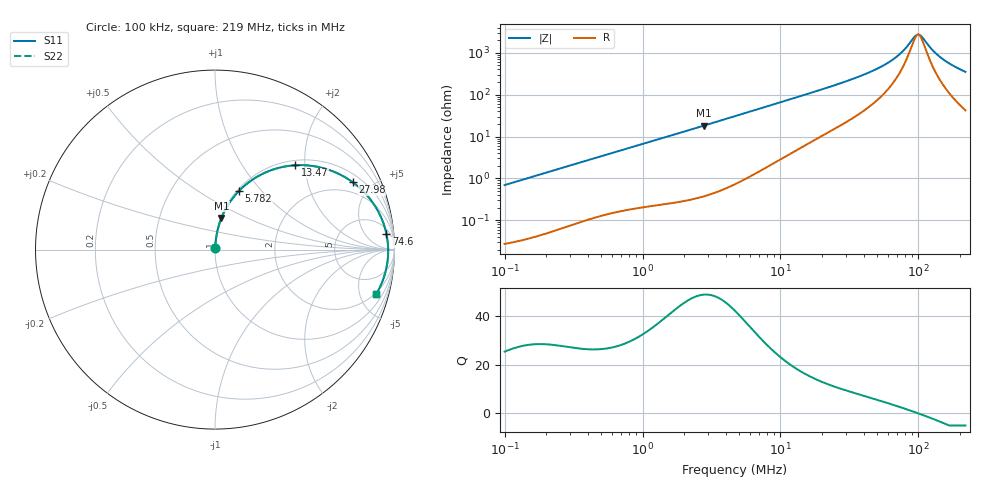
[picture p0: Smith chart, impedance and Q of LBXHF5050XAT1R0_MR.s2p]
! LBXHF5050XAT1R0_MR  S-PARAMETER MODEL  ( General Type )
! Model Generated by TAIYO YUDEN Corporation (http://www.ty-top.com)
! Version 1.0
! TAIYO YUDEN Control No. 201118NI43SB-FBB
! Copyright(c) 2020 TAIYO YUDEN CO.,LTD. All Rights Reserved.
! Product Description (link to TY-COMPAS)
! https://ds.yuden.co.jp/TYCOMPAS/or/detail?pn=LBXHF5050XAT1R0NMR&u=M
! Products Name : Inductors
! Characteristics :
!  Inductance : 1.0 uH , SRF(min) : 85 MHz , DC Resistance(max) : 0.0185 Ohm
!  Rated Current : Saturation :7500 mA , Temp Rise : 3100 mA
!  Case Size : 5.0 x 5.0 / 0.197 x 0.197 [mm/inch] , Thickness : 3.1 / 0.122 [mm/inch]
!  (Conditions: Temperature = 25 degC , DC Bias Current/Voltage = 0A / 0V)
! External Node Assignments :
!  1  o---GGG---o  2
! GND o---------o GND
! Frequency Range : 0.1MHz  -  218.972167MHz  [ 402 STEP ]
# MHz S RI R 50
! Freq[MHz].  S11 Real  S11 Imag  S21 Real  S21 Imag  S12 Real  S12 Imag  S22 Real  S22 Imag
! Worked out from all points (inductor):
!   401 points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, 100 kHz to 219 MHz, reference 50 ohm
!   read as one part in series: L = 1.1 uH near 103.9 kHz
!   highest Q = 48.8 at 2.784 MHz (marker M1), where L = 1.04 uH
!   self-resonance near 99.47 MHz
!   S11 on the Smith chart (normalised r, x): 100 kHz: 1.00, +0.01; 5.782 MHz: 1.02, +0.76; 13.47 MHz: 1.10, +1.78; 27.98 MHz: 1.39, +3.85; 74.6 MHz: 8, +18; 219 MHz: 1.85, -6.98
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0.1  0.000322 0.00694  0.9997 -0.00694  0.9997 -0.00694  0.000322 0.00694
0.362673  0.00154 0.0246  0.9985 -0.0246  0.9985 -0.0246  0.00154 0.0246
1.315317  0.00973 0.0857  0.9903 -0.0857  0.9903 -0.0857  0.00973 0.0857
2.784314  0.0357 0.1756  0.9643 -0.1756  0.9643 -0.1756  0.0357 0.1756
4.770297  0.0951 0.2817  0.9049 -0.2817  0.9049 -0.2817  0.0951 0.2817
5.781695  0.1332 0.3264  0.8668 -0.3264  0.8668 -0.3264  0.1332 0.3264
8.658159  0.2541 0.4167  0.7459 -0.4167  0.7459 -0.4167  0.2541 0.4167
13.47404  0.4468 0.4699  0.5532 -0.4699  0.5532 -0.4699  0.4468 0.4699
16.97108  0.5577 0.4639  0.4423 -0.4639  0.4423 -0.4639  0.5577 0.4639
27.97917  0.7674 0.3751  0.2326 -0.3751  0.2326 -0.3751  0.7674 0.3751
43.54189  0.8874 0.2495  0.1126 -0.2495  0.1126 -0.2495  0.8874 0.2495
61.54953  0.9394 0.1443  0.0606 -0.1443  0.0606 -0.1443  0.9394 0.1443
74.59925  0.9554 0.0862  0.0446 -0.0862  0.0446 -0.0862  0.9554 0.0862
82.12764  0.9604 0.0574  0.0396 -0.0574  0.0396 -0.0574  0.9604 0.0574
93.96068  0.9643 0.0171  0.0357 -0.0171  0.0357 -0.0171  0.9643 0.0171
97.64457  0.9647 0.00555  0.0353 -0.00555  0.0353 -0.00555  0.9647 0.00555
101.4729  0.9649 -0.00599  0.0351 0.00599  0.0351 0.00599  0.9649 -0.00599
107.4986  0.9646 -0.0233  0.0354 0.0233  0.0354 0.0233  0.9646 -0.0233
127.8091  0.9598 -0.0758  0.0402 0.0758  0.0402 0.0758  0.9598 -0.0758
143.4391  0.9531 -0.1113  0.0469 0.1113  0.0469 0.1113  0.9531 -0.1113
173.851  0.935 -0.1716  0.065 0.1716  0.065 0.1716  0.935 -0.1716
218.9722  0.8997 -0.2457  0.1003 0.2457  0.1003 0.2457  0.8997 -0.2457
